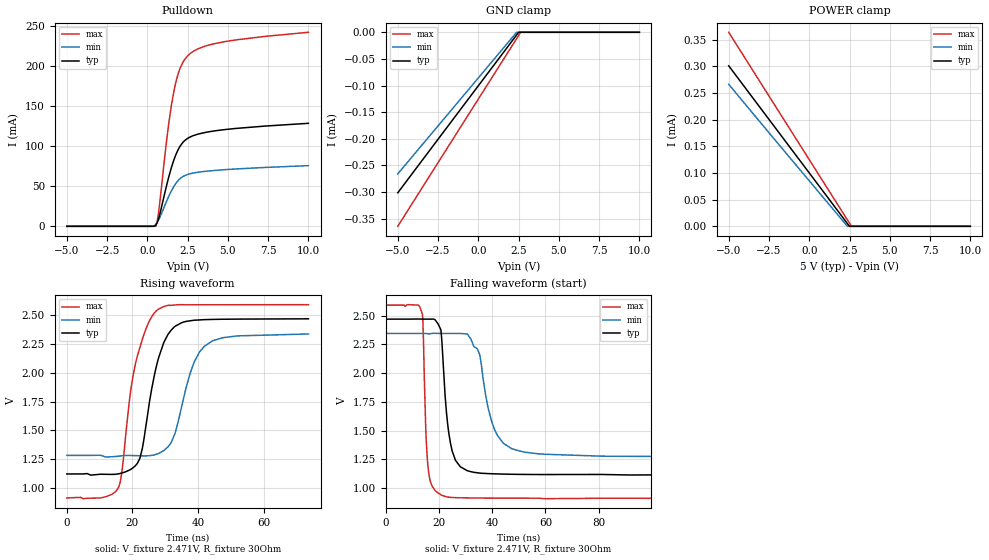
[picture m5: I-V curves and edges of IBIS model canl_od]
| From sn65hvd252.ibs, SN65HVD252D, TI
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|   canl_od Model
[Model]   canl_od
Model_type   Open_drain
Polarity   Non-Inverting
Vmeas = 1.8
Vref = 2.471
Cref = 100pF
Rref = 30
|   typ   min   max
|   (nom PVT)   (fast PVT)   (slow PVT)
C_comp   1.042e-11   8.984e-12   1.478e-11
| Where nom  PVT is Nominal Process, 5V, 27C
|   Fast PVT is Strong Process,  5.25V, -40C
|   Slow PVT is Weak Process,   4.75V, 125C
[Voltage Range]   5   4.75   5.25
|Ambient Temperature   25   85   -40
|Junction Temperature
[Temperature Range]   27   125   -40
[Pullup Reference]   5   4.75   5.25
[Pulldown Reference]   0   0   0
[Power Clamp Reference]   5   4.75   5.25
[GND Clamp Reference]   0   0   0
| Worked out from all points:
|   slope of the pulldown table from 0 to 0.75 V, typ, clamps not added: 56 ohm
|   falling waveform, V_fixture 2.471V, R_fixture 30Ohm: 20-80 % time 3.03ns typ, 5.7ns min, 1.44ns max; typ from 2.47 V to 1.12 V
|   rising waveform, V_fixture 2.471V, R_fixture 30Ohm: 20-80 % time 5.49ns typ, 6.26ns min, 5.43ns max; typ from 1.12 V to 2.47 V
[Pulldown]
|   Voltage   I(typ)   I(min)   I(max)
-5V       0A         0A         0A
334.2mV   1.748uA    71.49uA    22.32nA
533.5mV   1.851mA    2.947mA    736.8uA
612.2mV   4.915mA    5.15mA     6.734mA
712mV     10.62mA    8.57mA     20.03mA
1.305V    59.9mA     36.49mA    125mA
1.647V    82.95mA    49.82mA    168.6mA
2.035V    100.2mA    59.6mA     197.6mA
2.6V      111mA      65.41mA    214.8mA
3.594V    117.2mA    68.68mA    225.1mA
4.902V    121mA      70.88mA    231mA
10V       128.7mA    75.79mA    242.4mA
[GND Clamp]
|   Voltage   I(typ)   I(min)   I(max)
-5V       -301.3uA   -265.7uA   -364.2uA
2.377V    -5.104uA   -90.53nA   -12.01uA
2.51V     0A         0A         -5.653uA
2.628V    0A         0A         -15.1nA
10V       0A         0A         0A
[POWER Clamp]
|   Voltage   I(typ)   I(min)   I(max)
-5V       301uA      266.4uA    363.9uA
2.367V    5.163uA    125.4nA    12.12uA
2.495V    39.33nA    0A         6.028uA
2.618V    0A         0A         175.6nA
10V       0A         0A         0A
[Ramp]
R_load = 30
|   typ   min   max
dV/dt_r   0.809782/5.44848e-09   0.637809/6.27035e-09   1.00805/5.4242e-09
dV/dt_f   0.809828/3.016e-09   0.638062/5.62224e-09   1.00806/1.43891e-09
[Falling Waveform]
V_fixture = 2.471V
V_fixture_min = 2.346V
V_fixture_max = 2.593V
R_fixture = 30Ohm
|   Time   V(typ)   V(min)   V(max)
0s        2.471V     2.346V     2.593V
13.8ns    2.471V     2.346V     2.513V
15.8ns    2.471V     2.344V     1.204V
21.2ns    2.237V     2.346V     935.8mV
24.3ns    1.392V     2.346V     918.7mV
30.7ns    1.15V      2.34V      913.8mV
35.3ns    1.13V      2.159V     912.5mV
40.9ns    1.123V     1.508V     911.6mV
47.3ns    1.12V      1.343V     911.5mV
181.1ns   1.12V      1.28V      912.3mV
[Rising Waveform]
V_fixture = 2.471V
V_fixture_min = 2.346V
V_fixture_max = 2.593V
R_fixture = 30Ohm
|   Time   V(typ)   V(min)   V(max)
0s        1.121V     1.283V     912.9mV
15.7ns    1.122V     1.275V     1.002V
16.8ns    1.13V      1.279V     1.143V
20.8ns    1.19V      1.281V     2.062V
23ns      1.34V      1.279V     2.288V
27.7ns    2.1V       1.296V     2.548V
31.8ns    2.37V      1.393V     2.586V
37.6ns    2.452V     1.994V     2.591V
41.9ns    2.462V     2.229V     2.591V
73.7ns    2.469V     2.337V     2.592V
